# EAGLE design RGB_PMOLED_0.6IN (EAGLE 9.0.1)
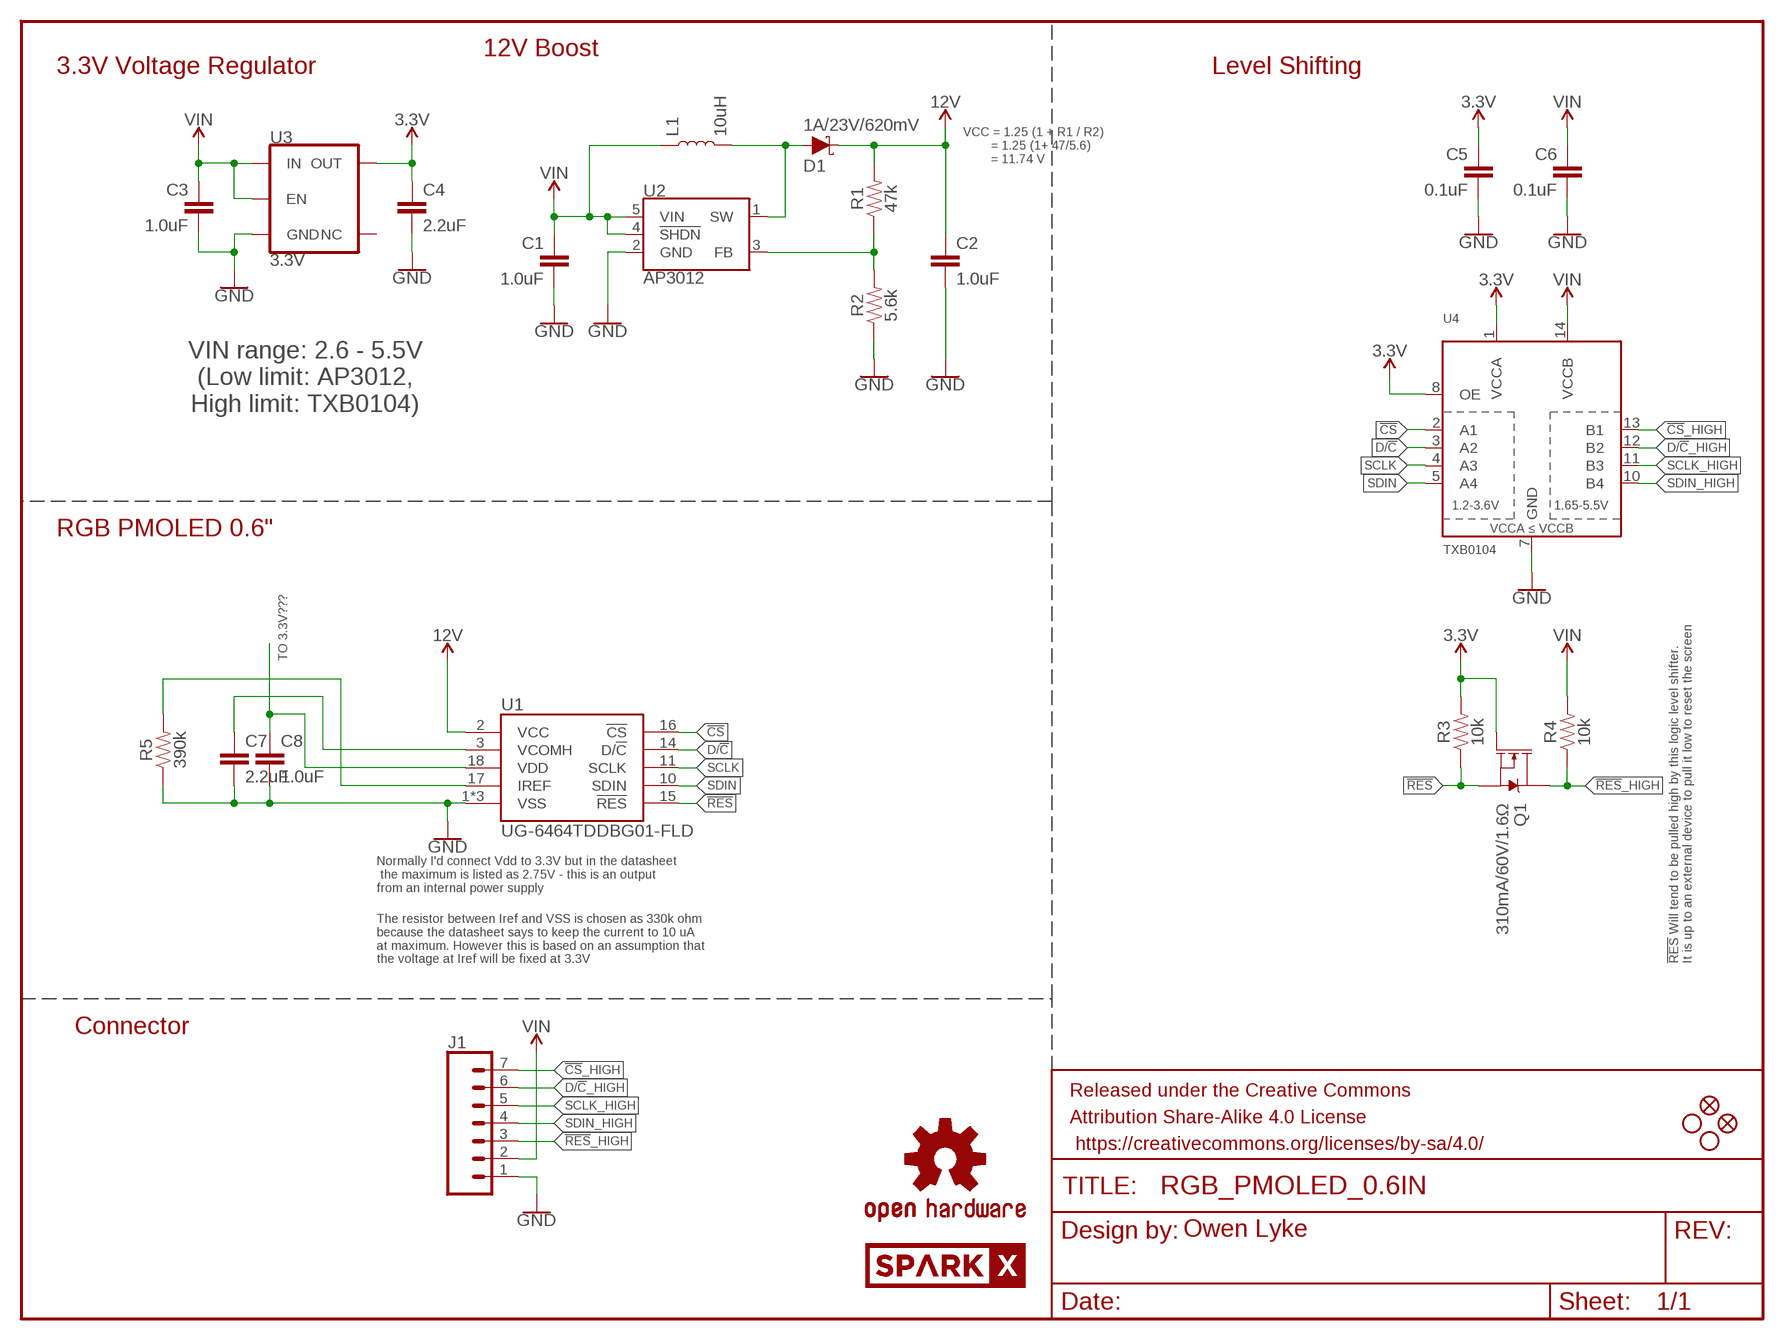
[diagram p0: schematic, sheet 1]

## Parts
C1  1.0uF  1.0UF-0603-16V-10%  [0603]
C2  1.0uF  1.0UF-0603-16V-10%  [0603]
C3  1.0uF  1.0UF-0603-16V-10%  [0603]
C4  2.2uF  2.2UF-0603-10V-20%  [0603]
C5  0.1uF  0.1UF-0603-25V-(+80/-20%)  [0603]
C6  0.1uF  0.1UF-0603-25V-(+80/-20%)  [0603]
C7  2.2uF  2.2UF-0805-25V-(+80/-20%)  [0805]
C8  1.0uF  1.0UF-0603-16V-10%  [0603]
D1  1A/23V/620mV  DIODE-SCHOTTKY-BAT20J  [SOD-323]
FD1  FIDUCIAL1X2  [FIDUCIAL-1X2]
FD2  FIDUCIAL1X2  [FIDUCIAL-1X2]
FRAME1  FRAME-LETTER  [CREATIVE_COMMONS]
H1  STAND-OFF  [STAND-OFF]
H2  STAND-OFF  [STAND-OFF]
J1  CONN_07NO_SILK  [1X07_NO_SILK]
L1  10uH  INDUCTORINDUCTOR_10UH  [INDUCTOR_3X3]
LOGO1  SPARKX-LOGO5  [SPARKX-LARGE]
LOGO2  OSHW-LOGOS  [OSHW-LOGO-S]
Q1  310mA/60V/1.6Ω  MOSFET-NCH-2N7002PW  [SOT323]
R1  47k  47KOHM-0603-1/10W-1%  [0603]
R2  5.6k  5.6KOHM-0603-1/10W-1%  [0603]
R3  10k  10KOHM-0603-1/10W-1%  [0603]
R4  10k  10KOHM-0603-1/10W-1%  [0603]
R5  390k  390KOHM-0603-1/10W-1%  [0603]
U1  UG-6464TDDBG01-FLD  [UG-6464TDDBG01-FOLDED]
U2  AP3012  [SOT23-5]
U3  3.3V  V_REG_AP2112K-3.3V  [SOT23-5]
U4  TXB0104  TXB0104PWRSOIC14  [SO14]

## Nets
3.3V: C4.1 C5.1 Q1.1(G) R3.2 U3.5(OUT) U4.1(VCCA) U4.8(OE)
12V: C2.1 D1.C R1.2 U1.2(VCC)
!CS: U1.16(!CS) U4.2(A1)
!CS!_HIGH: J1.7 U4.13(B1)
!RES: Q1.2(S) R3.1 U1.15(!RES)
!RES!_HIGH: J1.3 Q1.3(D) R4.1
D/!C: U1.14(D/!C) U4.3(A2)
D/!C!_HIGH: J1.6 U4.12(B2)
GND: C1.2 C2.2 C3.2 C4.2 C5.2 C6.2 C7.2 C8.2 J1.1 R2.1 R5.1 U1.1(VSS) U1.19(VSS) U1.20(VSS) U2.2(GND) U3.2(GND) U4.7(GND)
N$2: D1.A L1.P$2 U2.1(SW)
N$3: R1.1 R2.2 U2.3(FB)
N$5: C7.1 U1.3(VCOMH)
N$10: C8.1 U1.18(VDD)
N$11: R5.2 U1.17(IREF)
SCLK: U1.11(SCLK) U4.4(A3)
SCLK_HIGH: J1.5 U4.11(B3)
SDIN: U1.10(SDIN) U4.5(A4)
SDIN_HIGH: J1.4 U4.10(B4)
VIN: C1.1 C3.1 C6.1 J1.2 L1.P$1 R4.2 U2.4(!SHDN!) U2.5(VIN) U3.1(IN) U3.3(EN) U4.14(VCCB)
Unconnected: U3.4(NC)

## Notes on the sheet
- 12V Boost
- 3.3V Voltage Regulator | Level Shifting
- VCC = 1.25 (1 + R1 / R2)
          = 1.25 (1+ 47/5.6)
          = 11.74 V
- VIN range: 2.6 - 5.5V
  (Low limit: AP3012,
  High limit: TXB0104)
- RGB PMOLED 0.6"
- TO 3.3V???
- Normally I'd connect Vdd to 3.3V but in the datasheet
   the maximum is listed as 2.75V - this is an output 
  from an internal power supply
- The resistor between Iref and VSS is chosen as 330k ohm 
  because the datasheet says to keep the current to 10 uA 
  at maximum. However this is based on an assumption that 
  the voltage at Iref will be fixed at 3.3V
- !RES! Will tend to be pulled high by this logic level shifter. 
  It is up to an external device to pull it low to reset the screen
- Connector
- Owen Lyke

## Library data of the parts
C1-C3 C8 = SparkFun-Capacitors:1.0UF: 1µF ceramic capacitors; PROD_ID: CAP-00868
C4 = SparkFun-Capacitors:2.2UF: 2.2µF ceramic capacitors; PROD_ID: CAP-07888
C5 C6 = SparkFun-Capacitors:0.1UF: 0.1µF ceramic capacitors; PROD_ID: CAP-00810
C7 = SparkFun-Capacitors:2.2UF: 2.2µF ceramic capacitors; PROD_ID: CAP-11624
D1 = SparkFun-DiscreteSemi:DIODE-SCHOTTKY: Schottky diode; PROD_ID: DIO-11623
FD1 FD2 = SparkFun-Aesthetics:FIDUCIAL: Fiducial Alignment Points
FRAME1 = SparkFun-Aesthetics:FRAME-LETTER: Schematic Frame - Letter
H1 H2 = SparkFun-Hardware:STAND-OFF: Stand Off
J1 = SparkFun-Connectors:CONN_07: Multi connection point. Often used as Generic Header-pin footprint for 0.1 inch spaced/style header connections On any of the 0.1 inch spaced packages, you can populate with these: Break Away Headers - Straight (PRT-00116) Break Away Male Headers - Right Angle (PRT-00553) Female Headers (PRT-00115)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
L1 = 1.81_Greyscale_OLED_Breakout:INDUCTOR: Inductors
LOGO1 = 1.81_Greyscale_OLED_Breakout:SPARKX-LOGO
LOGO2 = SparkFun-Aesthetics:OSHW-LOGO: Open-Source Hardware (OSHW) Logo
Q1 = SparkFun-DiscreteSemi:MOSFET-NCH: N-channel MOSFETs Voltage controlled devices that allow control of high current outputs. SparkFun Products: SparkFun OpenScale SparkFun Digital Sandbox SparkFun Monster Moto Shield SparkFun MOSFET Power Controller; PROD_ID: TRANS-11151
R1 = SparkFun-Resistors:47KOHM: 47kΩ resistor; PROD_ID: RES-07871
R2 = SparkFun-Resistors:5.6KOHM: 5.6kΩ resistor; PROD_ID: RES-12378
R3 R4 = SparkFun-Resistors:10KOHM: 10kΩ resistor; PROD_ID: RES-00824
R5 = SparkFun-Resistors:390KOHM: 390kΩ resistor; PROD_ID: RES-12024
U1 = RGB_OLED:UG-6464TDDBG01
U2 = 1.81_Greyscale_OLED_Breakout:AP3012: AP3012 The AP3012 is a high power, constant frequency, current mode PWM, inductor based, step-up (boost) converter. The converter operates at high frequency (1.5MHz) so that a small, low profile inductor can be used. Datasheet
U3 = SparkFun-IC-Power:V_REG_AP2112: AP2112 - 600mA CMOS LDO Regulator w/ Enable The AP2112 is CMOS process low dropout linear regulator with enable function, the regulator delivers a guaranteed 600mA (min.) continuous load current. Features Output Voltage Accuracy: ±1.5% Output Current: 600mA (Min.) Foldback Short Current Protection: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; PROD_ID: VREG-12457
U4 = SparkFun-IC-Comms:TXB0104PWR: 4-Bit Bi-Directional Level Shifter 1.2V-3.6V (VCCA) to 1.65V-5.5V (VCCB) bi-directional level shifter with auto direction sensing. Max data rate - VCCA 1.8V: 20Mbps (50ns), VCCA 3.3V: 100Mbps (10ns) Digikey: 296-21929-1-ND (TSSOP) Datasheet SparkFun Products SparkFun Cellular Shield - MG2639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; PROD_ID: IC-11329

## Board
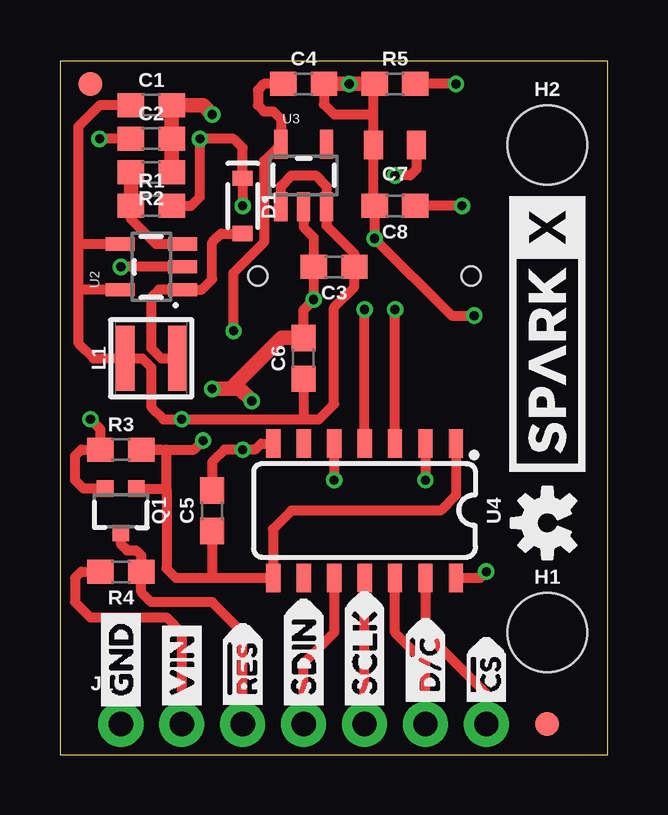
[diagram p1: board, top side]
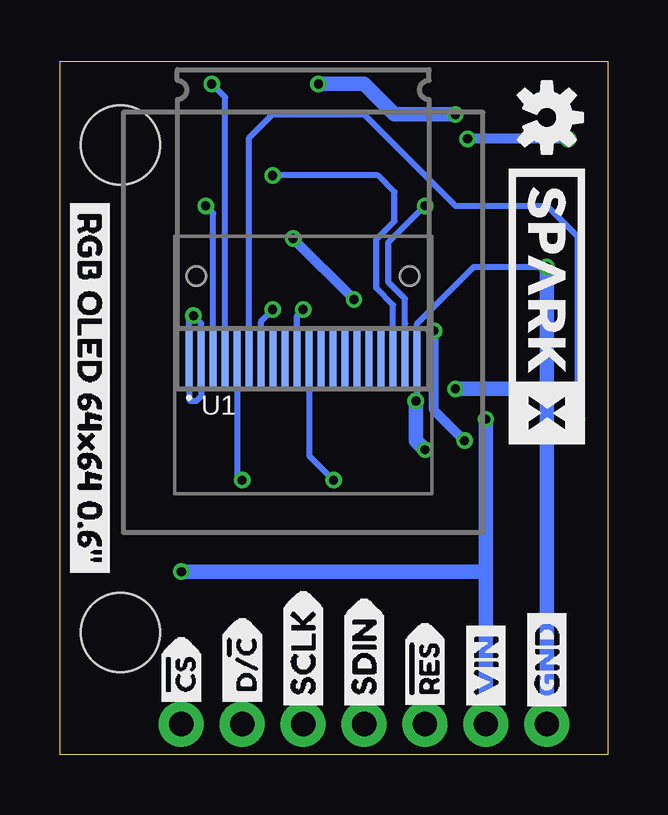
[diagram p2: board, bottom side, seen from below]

Size 22.84 x 28.88 mm. Coordinates in mm from the lower left corner, seen from the top.
Outline: 0,0 22.84,0 22.84,28.88 0,28.88 0,0
Copper layers (1*16): Top 0.035mm / dielectric 1.5mm / Bottom 0.035mm
Design rules "SparkFun-2-layer-PCBWay-LIMIT": minimum track width 6mil, minimum drill 0.3mm, track to track 6mil, track to pad 6mil, pad to pad 6mil, via to via 6mil, smd to smd 6mil, copper to edge 6mil, drill to drill 6mil, minimum pad ring 6mil, minimum via ring 6mil, stop-mask expansion 4mil, vias tented up to drill 25mil, thermal gap 10mil

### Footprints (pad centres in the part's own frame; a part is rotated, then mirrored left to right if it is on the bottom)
0603 = smd 1.1 x 1: 1 -0.85,0; 2 0.85,0
0805 = smd 0.8 x 1.2: 1 -0.9,0; 2 0.9,0
SOD-323 = smd 0.63 x 0.83: A 1.15,0; C -1.15,0
FIDUCIAL-1X2 = smd 1 x 1: 1 0,0
STAND-OFF = hole 3.302: 0,0
1X07_NO_SILK = drill 1.016 pad 1.88: 1 0,0; 2 2.54,0; 3 5.08,0; 4 7.62,0; 5 10.16,0; 6 12.7,0; 7 15.24,0
INDUCTOR_3X3 = smd 2.7 x 0.8: P$1 0,1.1; P$2 0,-1.1
SOT323 = smd 0.7 x 0.7: 1 -0.65,-0.925; 2 0.65,-0.925; 3 0,0.925
UG-6464TDDBG01-FOLDED = smd 0.3 x 2.5: 1 4.75,1.25; 2 4.25,1.25; 3 3.75,1.25; 4 3.25,1.25; 5 2.75,1.25; 6 2.25,1.25; 7 1.75,1.25; 8 1.25,1.25; 9 0.75,1.25; 10 0.25,1.25; 11 -0.25,1.25; 12 -0.75,1.25; 13 -1.25,1.25; 14 -1.75,1.25; 15 -2.25,1.25; 16 -2.75,1.25; 17 -3.25,1.25; 18 -3.75,1.25; 19 -4.25,1.25; 20 -4.75,1.25 | hole 0.8: -4.45,4.7; 4.45,4.7
SOT23-5 = smd 0.55 x 1.2: 1 -0.95,-1.3; 2 0,-1.3; 3 0.95,-1.3; 4 0.95,1.3; 5 -0.95,1.3
SO14 = smd 0.6 x 1.2: 1 -3.81,-2.8; 2 -2.54,-2.8; 3 -1.27,-2.8; 4 0,-2.8; 5 1.27,-2.8; 6 2.54,-2.8; 7 3.81,-2.8; 8 3.81,2.8; 9 2.54,2.8; 10 1.27,2.8; 11 0,2.8; 12 -1.27,2.8; 13 -2.54,2.8; 14 -3.81,2.8

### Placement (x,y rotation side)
C1  3.81,27.05 0 top
C2  3.81,25.65 0 top
C3  11.43,20.32 180 top
C4  10.16,27.94 0 top
C5  6.35,10.16 90 top
C6  10.16,16.51 90 top
C7  13.97,25.4 180 top
C8  13.97,22.86 180 top
D1  7.62,22.86 270 top
FD1  1.27,27.94 0 top
FD2  20.32,1.27 0 top
FRAME1  not placed on the board
H1  20.32,5.08 0 top
H2  20.32,25.4 0 top
J1  2.54,1.27 0 top
L1  3.81,16.51 90 top
LOGO1  20.32,17.53 90 top
LOGO2  20.32,9.65 90 top
LOGO3  SPARKX-LOGO5  [SPARKX-LARGE]  2.54,18.67 270 bottom
LOGO4  OSHW-LOGOS  [OSHW-LOGO-S]  2.54,26.54 270 bottom
Q1  2.54,10.16 180 top
R1  3.81,22.86 0 top
R2  3.81,24.26 180 top
R3  2.54,12.7 0 top
R4  2.54,7.62 180 top
R5  13.97,27.94 0 top
U1  12.7,15.24 0 bottom
U2  3.81,20.32 90 top
U3  10.16,24.13 0 top
U4  12.7,10.16 180 top
U$1  [VIN0]  5.08,1.52 90 top
U$2  [VIN0]  5.08,1.52 90 bottom
U$3  [SDIN3]  10.16,1.52 90 top
U$4  [SDIN3]  10.16,1.52 90 bottom
U$5  [SCLK4]  12.7,1.52 90 top
U$6  [SCLK4]  12.7,1.52 90 bottom
U$7  [GND1]  2.54,1.52 90 top
U$8  [GND1]  2.54,1.52 90 bottom
U$9  [D##C5]  15.24,1.52 90 top
U$10  [#RES2]  7.62,1.4 90 top
U$11  [#RES2]  7.62,1.4 90 bottom
U$12  [#CS6]  17.78,1.52 90 top
U$13  [#CS6]  17.78,1.52 90 bottom
U$14  [D##C5]  15.24,1.52 90 bottom
U$16  [RGB_OLED_64X64_0#6#7]  21.59,23.5 270 bottom

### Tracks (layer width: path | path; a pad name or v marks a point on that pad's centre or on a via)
3.3V  (via drill 0.38)
  Top 0.406: C4.1 8.51,27.94 8.26,27.69 8.26,27.05 8.51,26.8 8.89,26.8 9.21,26.48 U3.5 8.51,24.73 8.51,21.34 7.24,20.07 v7.24,17.65 | 4.19,12.7 R3.2 4.45,12.7 | U4.8 | U4.1 16.51,10.79 15.88,10.16 9.65,10.16 8.88,9.39 U4.8 | 4.45,11.05 4.45,7.75 4.83,7.37 6.22,7.37 | 6.22,7.37 U4.8 | Q1.1 4.41,11.09 4.45,11.05 | C5.1 6.35,7.49 6.22,7.37 | 4.45,12.7 5.59,12.7 v5.97,13.08 | 4.45,11.05 4.45,12.7
  Bottom 0.406: v5.97,13.08 7.24,14.35 v7.24,17.65
12V  (via drill 0.38)
  Top 0.406: C2.1 v1.65,25.65 | v7.62,22.86 D1.C 7.62,25.27 7.24,25.65 v5.84,25.65 5.84,23.24 5.46,22.86 R1.2
  Bottom 0.254: 8.45,17.96 U1.2 8.45,18.99 9.14,19.68 9.14,21.34 v7.62,22.86
  Bottom 0.406: v1.65,25.65 v5.84,25.65
!CS  (via drill 0.38)
  Top 0.406: U4.2 v15.24,11.43
  Bottom 0.254: U1.16 15.45,11.64 v15.24,11.43
!CS!_HIGH
  Top 0.406: J1.7 17.78,2.54 15.24,5.08 U4.13
!RES  (via drill 0.38)
  Top 0.406: Q1.2 0.98,11.09 0.64,11.43 0.64,12.45 0.89,12.7 R3.1 1.69,13.55 v1.27,13.97
  Bottom 0.254: v1.27,13.97 1.27,21.59 2.54,22.86 6.35,22.86 10.16,26.67 13.97,26.67 14.95,25.69 U1.15
!RES!_HIGH
  Top 0.406: Q1.3 2.54,8.76 2.79,8.51 3.17,8.51 3.39,8.29 R4.1 3.39,6.77 3.81,6.35 6.35,6.35 7.62,5.08 J1.3
D/!C  (via drill 0.38)
  Top 0.406: U4.3 v13.97,18.54
  Bottom 0.254: U1.14 14.45,18.06 v13.97,18.54
D/!C!_HIGH
  Top 0.406: J1.6 15.24,3.81 13.97,5.08 U4.12
GND  (via drill 0.38)
  Top 0.406: C6.2 10.16,18.54 v10.58,18.96 C3.2 10.58,21.55 10.16,21.97 U3.2 | 13.07,26.67 C7.2 13.07,22.91 C8.2 v13.12,21.5 16.33,18.29 v17.27,18.29 | 13.07,26.67 13.07,27.89 R5.1 | C4.2 11.01,27.09 11.43,26.67 13.07,26.67 | C5.2 6.35,12.19 6.86,12.7 v7.62,12.7 8.13,12.7 8.39,12.96 U4.7 | U2.2 v2.54,20.32
  Top 0.61: R2.1 C2.2 C1.2 5.97,27.05 v6.35,26.67 | C6.2 9.23,17.36 7.11,15.24 v6.35,15.24 7.49,15.24 v8,14.73 | C4.2 v12.06,27.94 R5.1
  Bottom 0.254: v2.54,20.32 5.59,20.32 7.95,17.96 U1.1 7.95,14.78 v8,14.73 | U1.19 16.95,14.93 17.14,14.73 17.4,14.73 17.45,14.78 U1.20 17.45,18.11 v17.27,18.29 16.95,17.97 U1.19
  Bottom 0.406: v10.58,18.96 v13.12,21.5
  Bottom 0.61: J1.1 2.54,15.24 | 2.54,15.24 v2.54,20.32 | v6.35,15.24 2.54,15.24 | v6.35,26.67 8.89,26.67 10.16,27.94 v12.06,27.94 | v8,14.73 8,13.08 v7.62,12.7
N$2
  Top 0.406: D1.A 6.72,21.71 6.35,21.34 6.35,19.81 5.91,19.37 U2.1 4.13,19.37 3.81,19.05 3.81,16.92 4.22,16.51 L1.P$2
N$3
  Top 0.406: U2.3 4,21.27 2.96,22.31 R1.1
  Top 0.61: R1.1 R2.2
N$5  (via drill 0.38)
  Top 0.406: C7.1 14.87,24.39 14.61,24.13 v13.97,24.13
  Bottom 0.254: v13.97,24.13 9.59,24.13 8.89,23.43 8.89,22.23 9.65,21.46 9.65,19.43 8.95,18.73 U1.3
N$10  (via drill 0.38)
  Top 0.406: v16.76,22.86 C8.1
  Bottom 0.254: U1.18 16.45,22.55 v16.76,22.86
N$11  (via drill 0.38)
  Top 0.406: v16.51,27.94 R5.2
  Bottom 0.254: U1.17 15.95,27.38 v16.51,27.94
SCLK  (via drill 0.38)
  Top 0.406: U4.4 v12.7,18.54
  Bottom 0.254: U1.11 12.95,18.29 v12.7,18.54
SCLK_HIGH
  Top 0.406: J1.5 U4.11
SDIN  (via drill 0.38)
  Top 0.406: U4.5 v11.43,11.43
  Bottom 0.254: U1.10 12.45,12.45 v11.43,11.43
SDIN_HIGH
  Top 0.406: J1.4 10.16,3.81 11.43,5.08 U4.10
VIN  (via drill 0.38)
  Top 0.406: C1.1 1.65,27.05 0.76,26.16 0.76,21.21 | U3.1 9.21,23.69 9.65,24.13 10.67,24.13 11.11,23.69 U3.3 11.11,22.04 12.28,20.87 C3.1 12.28,19.48 11.43,18.63 11.43,14.61 10.79,13.97 10.16,13.97 | U4.14 17.52,7.36 v17.78,7.62 | 2.44,21.34 U2.4 0.82,21.27 0.76,21.21 | R4.2 0.89,7.62 0.64,7.37 0.64,6.35 1.27,5.71 4.45,5.71 5.08,5.08 J1.2 | 0.76,21.21 0.76,19.43 | 0.76,19.43 0.76,17.14 1.4,16.51 L1.P$1 3.43,16.51 3.81,16.13 3.81,14.48 4.32,13.97 v5.08,13.97 10.16,13.97 | U2.5 0.82,19.37 0.76,19.43 | C6.1 10.16,13.97
  Bottom 0.61: 5.08,6.35 J1.2 5.08,7.62 | 5.08,7.62 v5.08,13.97 | v17.78,7.62 5.08,7.62

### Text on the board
tDocu: Owen Lyke

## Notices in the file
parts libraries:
SparkFun-Aesthetics: Licensing: Creative Commons ShareAlike 4.0 International - https://creativecommons.org/licenses/by-sa/4.0
SparkFun-Aesthetics: Released under the Creative Commons Attribution Share-Alike 4.0 License
SparkFun-Aesthetics: https://creativecommons.org/licenses/by-sa/4.0
